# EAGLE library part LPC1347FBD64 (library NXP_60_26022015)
32-bit ARM Cortex-M3 microcontroller; up to 64 kB flash; up to 12 kB SRAM; USB device; USART; EEPROM The LPC1315/16/17/45/46/47 are ARM Cortex-M3 based microcontrollers for embedded applications featuring a high level of integration and low power consumption. The ARM Cortex-M3 is a next generation core that offers system enhancements such as enhanced debug features and a higher level of support block integration. The LPC1315/16/17/45/46/47 operate at CPU frequencies of up to 72 MHz. The ARM Cortex-M3 CPU incorporates a 3-stage pipeline and uses a Harvard architecture with separate local instruction and data buses as well as a third bus for peripherals. The ARM Cortex-M3 CPU also includes an internal prefetch unit that supports speculative branching. Equipped with a highly flexible and configurable Full-Speed USB 2.0 device controller available on the LPC1345/46/47, this series brings unparalleled design flexibility and seamless integration to today’s demanding connectivity solutions. The peripheral complement of the LPC1315/16/17/45/46/47 includes up to 64 kB of flash memory, 8 kB or 10 kB of SRAM data memory, one Fast-mode Plus I 2 C-bus interface, one RS-485/EIA-485 USART with support for synchronous mode and smart card interface, two SSP interfaces, four general purpose counter/timers, an 8-channel, 12-bit ADC, and up to 51 general purpose I/O pins. AAL Eindhoven MK
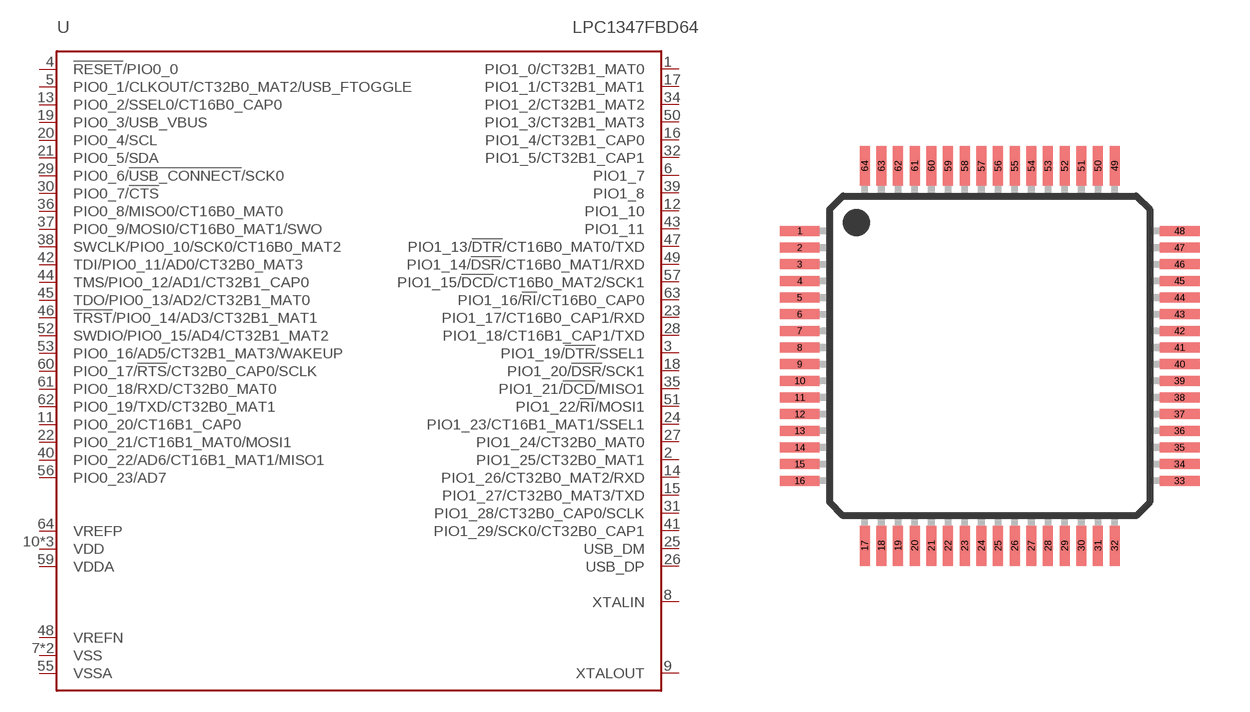
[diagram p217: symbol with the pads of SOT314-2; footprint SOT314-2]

Designator prefix U

## LPC1347FBD64 (EEPROM: 4kB; FLASH: 64kB; GPIO: 51; SRAM0: 8kB; SRAM1: 2kB; SRAM_USB: 2kB; USB: yes)  [SOT314-2]
1  PIO1_0/CT32B1_MAT0
2  PIO1_25/CT32B0_MAT1
3  PIO1_19/!DTR!/SSEL1
4  !RESET!/PIO0_0
5  PIO0_1/CLKOUT/CT32B0_MAT2/USB_FTOGGLE
6  PIO1_7
7  VSS  pwr
8  XTALIN  in
9  XTALOUT  out
10  VDD  pwr
11  PIO0_20/CT16B1_CAP0
12  PIO1_10
13  PIO0_2/SSEL0/CT16B0_CAP0
14  PIO1_26/CT32B0_MAT2/RXD
15  PIO1_27/CT32B0_MAT3/TXD
16  PIO1_4/CT32B1_CAP0
17  PIO1_1/CT32B1_MAT1
18  PIO1_20/!DSR!/SCK1
19  PIO0_3/USB_VBUS
20  PIO0_4/SCL
21  PIO0_5/SDA
22  PIO0_21/CT16B1_MAT0/MOSI1
23  PIO1_17/CT16B0_CAP1/RXD
24  PIO1_23/CT16B1_MAT1/SSEL1
25  USB_DM
26  USB_DP
27  PIO1_24/CT32B0_MAT0
28  PIO1_18/CT16B1_CAP1/TXD
29  PIO0_6/!USB_CONNECT!/SCK0
30  PIO0_7/!CTS!
31  PIO1_28/CT32B0_CAP0/SCLK
32  PIO1_5/CT32B1_CAP1
33  VDD  pwr
34  PIO1_2/CT32B1_MAT2
35  PIO1_21/!DCD!/MISO1
36  PIO0_8/MISO0/CT16B0_MAT0
37  PIO0_9/MOSI0/CT16B0_MAT1/SWO
38  SWCLK/PIO0_10/SCK0/CT16B0_MAT2
39  PIO1_8
40  PIO0_22/AD6/CT16B1_MAT1/MISO1
41  PIO1_29/SCK0/CT32B0_CAP1
42  TDI/PIO0_11/AD0/CT32B0_MAT3
43  PIO1_11
44  TMS/PIO0_12/AD1/CT32B1_CAP0
45  TDO/PIO0_13/AD2/CT32B1_MAT0
46  !TRST!/PIO0_14/AD3/CT32B1_MAT1
47  PIO1_13/!DTR!/CT16B0_MAT0/TXD
48  VREFN  pwr
49  PIO1_14/!DSR!/CT16B0_MAT1/RXD
50  PIO1_3/CT32B1_MAT3
51  PIO1_22/!RI!/MOSI1
52  SWDIO/PIO0_15/AD4/CT32B1_MAT2
53  PIO0_16/AD5/CT32B1_MAT3/WAKEUP
54  VSS  pwr
55  VSSA  pwr
56  PIO0_23/AD7
57  PIO1_15/!DCD!/CT16B0_MAT2/SCK1
58  VDD  pwr
59  VDDA  pwr
60  PIO0_17/!RTS!/CT32B0_CAP0/SCLK
61  PIO0_18/RXD/CT32B0_MAT0
62  PIO0_19/TXD/CT32B0_MAT1
63  PIO1_16/!RI!/CT16B0_CAP0
64  VREFP  pwr

## Footprint SOT314-2 (pad centres in mm)
SOT314-2 LQFP64: plastic low profile quad flat package; 64 leads; body 10 x 10 x 1.4 mm JEDEC: MS-026 IEC: 136E10
smd 1.2 x 0.3: 1 -5.7,3.75; 2 -5.7,3.25; 3 -5.7,2.75; 4 -5.7,2.25; 5 -5.7,1.75; 6 -5.7,1.25; 7 -5.7,0.75; 8 -5.7,0.25; 9 -5.7,-0.25; 10 -5.7,-0.75; 11 -5.7,-1.25; 12 -5.7,-1.75; 13 -5.7,-2.25; 14 -5.7,-2.75; 15 -5.7,-3.25; 16 -5.7,-3.75; 33 5.7,-3.75; 34 5.7,-3.25; 35 5.7,-2.75; 36 5.7,-2.25; 37 5.7,-1.75; 38 5.7,-1.25; 39 5.7,-0.75; 40 5.7,-0.25; 41 5.7,0.25; 42 5.7,0.75; 43 5.7,1.25; 44 5.7,1.75; 45 5.7,2.25; 46 5.7,2.75; 47 5.7,3.25; 48 5.7,3.75
smd 0.3 x 1.2: 17 -3.75,-5.7; 18 -3.25,-5.7; 19 -2.75,-5.7; 20 -2.25,-5.7; 21 -1.75,-5.7; 22 -1.25,-5.7; 23 -0.75,-5.7; 24 -0.25,-5.7; 25 0.25,-5.7; 26 0.75,-5.7; 27 1.25,-5.7; 28 1.75,-5.7; 29 2.25,-5.7; 30 2.75,-5.7; 31 3.25,-5.7; 32 3.75,-5.7; 49 3.75,5.7; 50 3.25,5.7; 51 2.75,5.7; 52 2.25,5.7; 53 1.75,5.7; 54 1.25,5.7; 55 0.75,5.7; 56 0.25,5.7; 57 -0.25,5.7; 58 -0.75,5.7; 59 -1.25,5.7; 60 -1.75,5.7; 61 -2.25,5.7; 62 -2.75,5.7; 63 -3.25,5.7; 64 -3.75,5.7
